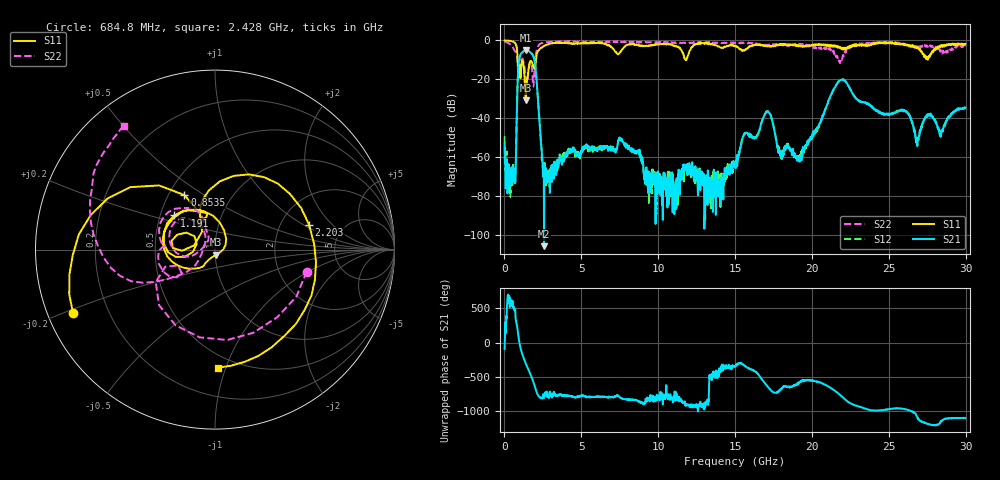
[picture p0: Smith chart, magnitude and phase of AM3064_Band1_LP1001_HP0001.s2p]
# Hz S DB R 50.0
!freq dBS11 angS11 dBS21 angS21 dBS12 angS12 dBS22 angS22
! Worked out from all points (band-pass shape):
!   1600 points, 10 MHz to 29.98 GHz, reference 50 ohm
!   highest |S21| = -4.85 dB at 1.397 GHz (marker M1); lowest = -105.9 dB at 2.578 GHz (marker M2)
!   |S21| within 3 dB of the highest: 1.018 GHz to 1.862 GHz (844.6 MHz wide, 58.6 % of centre)
!   lowest |S11| = -30.8 dB at 1.397 GHz (marker M3), VSWR 1.06, Z = 50.6 - j2.86 ohm
!   |S11| at or under -10 dB: 857.5 MHz to 2.047 GHz (1.189 GHz wide, 81.9 % of centre); 11.80399 GHz to 11.84059 GHz (36.6 MHz wide, 0.31 % of centre)
!   |S22| runs from -24.5 to -0.3 dB; largest |S21 - S12| = 0.0085
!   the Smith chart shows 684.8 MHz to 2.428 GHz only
!   S11 on the Smith chart (normalised r, x): 684.8 MHz: 0.08, -0.21; 853.5 MHz: 0.60, +0.42; 1.191 GHz: 0.59, +0.25; 2.203 GHz: 2.87, +1.13; 2.428 GHz: 0.40, -0.94
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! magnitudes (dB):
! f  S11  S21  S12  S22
! 10 MHz  0.0  -53.2  -49.4  -0.3
! 384.9 MHz  -0.3  -75.0  -80.6  -2.0
! 684.8 MHz  -1.3  -70.4  -69.5  -5.6
! 853.5 MHz  -9.2  -22.4  -22.2  -10.7
! 1.191 GHz  -10.6  -6.0  -5.9  -9.6
! 1.397 GHz  -30.8  -4.9  -4.9  -20.8
! 1.903 GHz  -13.8  -8.7  -8.7  -21.4
! 2.203 GHz  -5.3  -32.7  -32.6  -2.7
! 2.428 GHz  -3.6  -58.3  -61.6  -1.4
! 2.578 GHz  -2.8  -105.9  -67.7  -1.1
! 5.015 GHz  -1.5  -56.6  -57.7  -0.8
! 7.564 GHz  -5.7  -50.3  -51.1  -0.5
! 10 GHz  -2.0  -78.2  -73.8  -0.9
! 13.3 GHz  -1.7  -82.7  -70.5  -1.2
! 15 GHz  -3.0  -64.9  -64.6  -1.4
! 17.07 GHz  -2.9  -36.8  -36.7  -2.4
! 18 GHz  -2.0  -57.6  -58.8  -2.3
! 19.99 GHz  -2.7  -50.3  -49.4  -3.0
! 21.9 GHz  -4.3  -20.3  -20.2  -9.4
! 25 GHz  -1.1  -38.3  -38.0  -1.1
! 26.85 GHz  -4.1  -54.4  -53.7  -3.0
! 29.98 GHz  -1.8  -34.7  -34.7  -3.1
